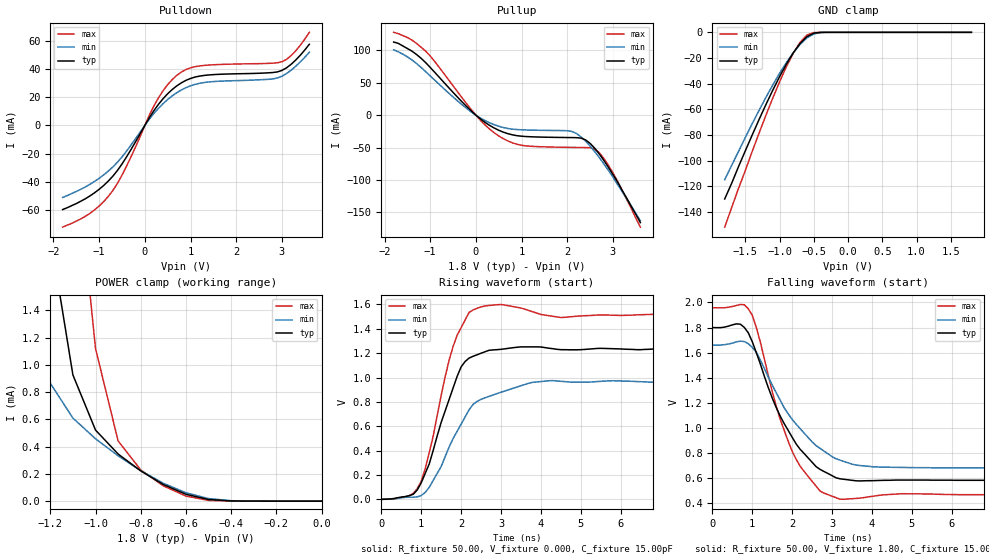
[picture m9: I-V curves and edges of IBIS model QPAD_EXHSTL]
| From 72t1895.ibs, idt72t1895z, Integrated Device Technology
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|   Model QPAD_EXHSTL
[Model]   QPAD_EXHSTL
Model_type   3-state
Polarity   Non-Inverting
Enable   Active-High
Vmeas =  0.900V
C_comp   3.00pF   NA   NA
[Temperature Range]   25.00   85.00   -40.00
[Voltage Range]   1.80V   1.60V   2.00V
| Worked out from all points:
|   slope of the pulldown table from 0 to 0.27 V, typ, clamps not added: 19.7 ohm
|   slope of the pullup table from 0 to 0.27 V, typ, clamps not added: 18.8 ohm
|   GND clamp passes 1 mA (typ) near -0.51 V on its own axis
|   POWER clamp passes 1 mA (typ) near -1.11 V on its own axis
|   rising waveform, R_fixture 50.00, V_fixture 0.000, C_fixture 15.00pF: 20-80 % time 731ps typ, 921ps min, 621ps max; typ from 0 V to 1.23 V
|   falling waveform, R_fixture 50.00, V_fixture 1.80, C_fixture 15.00pF: 20-80 % time 1.06ns typ, 1.22ns min, 854ps max; typ from 1.8 V to 0.579 V
[Pulldown]
| voltage   I(typ)   I(min)   I(max)
-1.8V     -59.8mA    -51.2mA    -72.3mA
-1.2V     -50.07mA   -41.81mA   -62.46mA
-700mV    -36.05mA   -29.51mA   -46.23mA
-400mV    -22.33mA   -18.22mA   -28.88mA
200mV     10.57mA    8.525mA    13.92mA
400mV     19.01mA    15.49mA    24.67mA
700mV     28.12mA    23.26mA    35.58mA
900mV     32.02mA    26.81mA    39.69mA
1.2V      35.04mA    29.92mA    42.26mA
3V        39.06mA    34.94mA    45.2mA
3.3V      46.36mA    41.95mA    52.89mA
3.6V      57.64mA    51.96mA    66.13mA
[Pullup]
| voltage   I(typ)   I(min)   I(max)
-1.8V     113mA      101mA      128mA
-1.4V     98.92mA    85.36mA    116mA
-1.1V     81.21mA    67.28mA    98.93mA
-100mV    6.412mA    4.931mA    8.552mA
500mV     -23.29mA   -17.11mA   -32.09mA
1V        -32.5mA    -22.61mA   -46.53mA
2.2V      -34.74mA   -28.29mA   -49.87mA
2.4V      -38.17mA   -40.02mA   -50.05mA
2.6V      -51.02mA   -56.23mA   -52.33mA
2.8V      -69.73mA   -75.15mA   -66.69mA
3.1V      -103mA     -107mA     -102mA
3.6V      -166mA     -163mA     -173mA
[GND_clamp]
| voltage   I(typ)   I(min)   I(max)
-1.8V     -130mA     -115mA     -152mA
-1.6V     -105mA     -93.09mA   -122mA
-1.3V     -68.22mA   -61mA      -78.85mA
-1.1V     -45.3mA    -41.22mA   -51.5mA
-1V       -34.68mA   -32.07mA   -38.72mA
-900mV    -24.85mA   -23.59mA   -26.87mA
-800mV    -16.08mA   -15.96mA   -16.35mA
-700mV    -8.721mA   -9.411mA   -7.76mA
-600mV    -3.357mA   -4.326mA   -2.135mA
-500mV    -667uA     -1.241mA   -218uA
-400mV    -58.99uA   -179uA     -9.374uA
1.8V      18.04nA    37.81nA    18nA
[POWER_clamp]
| voltage   I(typ)   I(min)   I(max)
-1.8V     20.11mA    12.65mA    31.29mA
-1.3V     3.744mA    1.476mA    8.598mA
-1.2V     1.95mA     866uA      5.327mA
-1.1V     927uA      610uA      2.766mA
-1V       522uA      458uA      1.121mA
-900mV    346uA      333uA      442uA
-800mV    222uA      224uA      229uA
-700mV    122uA      131uA      112uA
-600mV    50.35uA    61.27uA    37.19uA
-500mV    11.87uA    18.7uA     5.408uA
-400mV    1.361uA    3.089uA    377nA
0V        18.04nA    17.69nA    20nA
[Ramp]
| variable   typ   min   max
dV/dt_r   0.75/0.46n   0.58/0.56n   0.92/0.37n
dV/dt_f   0.74/0.69n   0.61/0.78n   0.89/0.57n
R_load = 50.00
[Rising Waveform]
R_fixture = 50.00
V_fixture = 0.000
C_fixture = 15.00pF
R_dut = 0.75
L_dut = 8.10nH
C_dut = 0.53pF
| time   V(typ)   V(min)   V(max)
0s        0V         0V         0V
700ps     30.4mV     17.21mV    30.27mV
1ns       136mV      31.04mV    148mV
1.5ns     632mV      270mV      854mV
1.8ns     916mV      500mV      1.257V
2ns       1.088V     618mV      1.41V
2.3ns     1.175V     780mV      1.555V
3ns       1.232V     880mV      1.6V
4.2ns     1.241V     974mV      1.508V
9.9ns     1.233V     968mV      1.514V
[Falling Waveform]
R_fixture = 50.00
V_fixture = 1.80
C_fixture = 15.00pF
R_dut = 0.75
L_dut = 8.10nH
C_dut = 0.53pF
| time   V(typ)   V(min)   V(max)
0s        1.8V       1.66V      1.958V
700ps     1.827V     1.691V     1.984V
1ns       1.687V     1.641V     1.898V
1.6ns     1.161V     1.279V     1.172V
2ns       923mV      1.066V     811mV
2.3ns     793mV      956mV      650mV
2.8ns     649mV      812mV      476mV
3.2ns     591mV      740mV      428mV
4.1ns     577mV      686mV      455mV
9.9ns     579mV      678mV      465mV
